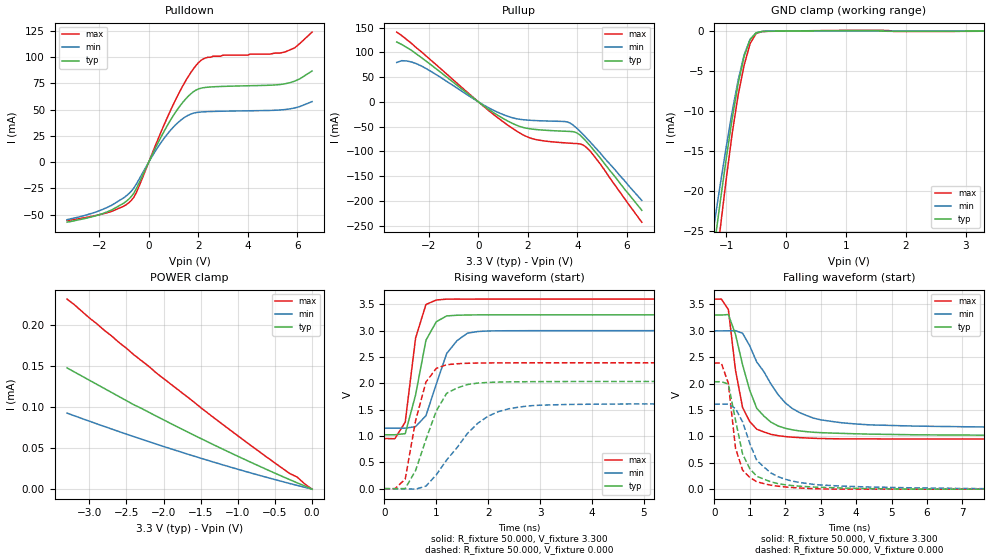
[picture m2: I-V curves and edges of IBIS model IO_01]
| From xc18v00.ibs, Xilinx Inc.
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|   Model IO_01
[Model]   IO_01
Model_type   I/O
Polarity   Inverting
Enable   Active-High
Vinl =   0.800V
Vinh =   2.000V
Vmeas =   1.650V
Cref =  50.000pF
Rref =   1.000M
Vref =  0.000V
C_comp   6.700pF   5.700pF   7.600pF
[Temperature Range]   50.000   100.000   0.000
[Voltage Range]   3.300V   3.000V   3.600V
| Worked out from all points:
|   slope of the pulldown table from 0 to 0.495 V, typ, clamps not added: 20.7 ohm
|   slope of the pullup table from 0 to 0.495 V, typ, clamps not added: 27.8 ohm
|   GND clamp passes 1 mA (typ) near -0.59 V on its own axis
|   rising waveform, R_fixture 50.000, V_fixture 3.300: 20-80 % time 297ps typ, 408ps min, 239ps max; typ from 1.02 V to 3.3 V
|   rising waveform, R_fixture 50.000, V_fixture 0.000: 20-80 % time 469ps typ, 827ps min, 316ps max; typ from 0 V to 2.04 V
|   falling waveform, R_fixture 50.000, V_fixture 3.300: 20-80 % time 642ps typ, 1.14ns min, 392ps max; typ from 3.3 V to 1.02 V
|   falling waveform, R_fixture 50.000, V_fixture 0.000: 20-80 % time 482ps typ, 780ps min, 329ps max; typ from 2.04 V to 0 V
[Pulldown]
| voltage   I(typ)   I(min)   I(max)
-3.3V     -57.2mA    -54.8mA    -55.7mA
-1.7V     -47.57mA   -43.39mA   -48.32mA
-700mV    -32.66mA   -27.57mA   -36.39mA
-500mV    -25.26mA   -20.88mA   -29mA
300mV     14.82mA    11.72mA    17.61mA
900mV     40.85mA    30.95mA    50.29mA
1.6V      62.9mA     44.78mA    81.73mA
2.1V      70.46mA    47.8mA     96.79mA
3V        72.23mA    48.59mA    102mA
5.5V      74.68mA    50.15mA    105mA
5.9V      77.27mA    51.71mA    109mA
6.6V      86.93mA    57.76mA    124mA
[Pullup]
| voltage   I(typ)   I(min)   I(max)
-3.3V     121mA      79.65mA    141mA
-2.9V     110mA      82.69mA    126mA
-2.3V     89.33mA    72.44mA    101mA
300mV     -11.04mA   -8.824mA   -12.73mA
1.5V      -46.27mA   -33.63mA   -57.51mA
1.9V      -52.76mA   -36.44mA   -68.97mA
2.3V      -55.67mA   -37.72mA   -75.79mA
3.7V      -59.69mA   -42.64mA   -83.42mA
4V        -63.32mA   -54.46mA   -84.35mA
4.2V      -71.44mA   -64.25mA   -86.4mA
4.5V      -87.94mA   -80.06mA   -98.42mA
6.6V      -219mA     -199mA     -243mA
[GND_clamp]
| voltage   I(typ)   I(min)   I(max)
-3.3V     -155mA     -140mA     -172mA
-1.2V     -26.97mA   -24.12mA   -31.21mA
-1.1V     -21.35mA   -19.21mA   -24.73mA
-1V       -15.97mA   -14.5mA    -18.53mA
-900mV    -10.95mA   -10.08mA   -12.81mA
-800mV    -6.54mA    -6.125mA   -7.981mA
-700mV    -3.156mA   -2.96mA    -4.255mA
-600mV    -1.062mA   -1.009mA   -1.564mA
-500mV    -216uA     -233uA     -293uA
-400mV    -48.58uA   -49.49uA   -64.66uA
700mV     37.32uA    20.73uA    65.45uA
3.3V      1.628nA    6.9uA      -17.62uA
[POWER_clamp]
| voltage   I(typ)   I(min)   I(max)
-3.3V     148uA      92.8uA     232uA
-2.4V     103uA      64.12uA    164uA
-1.5V     61.88uA    37.81uA    99.54uA
-500mV    19.51uA    11.69uA    31.91uA
-300mV    11.57uA    6.9uA      19.07uA
-200mV    7.689uA    4.565uA    14.73uA
-100mV    4uA        2.274uA    6.481uA
0V        1.628nA    6.511nA    380pA
[Ramp]
| variable   typ   min   max
dV/dt_r   1.221/0.443n   0.967/0.760n   1.433/0.321n
dV/dt_f   1.366/0.616n   1.101/1.088n   1.589/0.410n
R_load = 50.000
[Rising Waveform]
R_fixture = 50.000
V_fixture = 3.300
V_fixture_min = 3.000
V_fixture_max = 3.600
L_fixture = 0.000H
C_fixture = 0.000F
| time   V(typ)   V(min)   V(max)
0s        1.023V     1.148V     951mV
200ps     1.023V     1.148V     949mV
400ps     1.044V     1.148V     1.262V
600ps     1.779V     1.178V     2.859V
800ps     2.818V     1.386V     3.496V
1ns       3.169V     1.985V     3.581V
1.2ns     3.279V     2.566V     3.598V
1.6ns     3.297V     2.951V     3.598V
1.8ns     3.299V     2.983V     3.599V
10ns      3.299V     3V         3.599V
[Rising Waveform]
R_fixture = 50.000
V_fixture = 0.000
V_fixture_min = 0.000
V_fixture_max = 0.000
L_fixture = 0.000H
C_fixture = 0.000F
| time   V(typ)   V(min)   V(max)
0s        0V         0V         0V
200ps     -298uV     110uV      -3.088mV
400ps     1.188mV    -1.293mV   181mV
600ps     345mV      -9.507mV   1.291V
800ps     933mV      48.75mV    2.024V
1ns       1.477V     263mV      2.284V
1.2ns     1.811V     546mV      2.353V
1.8ns     2.004V     1.242V     2.385V
2.6ns     2.029V     1.549V     2.389V
10ns      2.035V     1.611V     2.389V
[Falling Waveform]
R_fixture = 50.000
V_fixture = 3.300
V_fixture_min = 3.000
V_fixture_max = 3.600
L_fixture = 0.000H
C_fixture = 0.000F
| time   V(typ)   V(min)   V(max)
0s        3.3V       3V         3.6V
200ps     3.299V     2.999V     3.602V
400ps     3.309V     3.001V     3.403V
600ps     2.934V     3.003V     2.257V
800ps     2.357V     2.955V     1.547V
1.2ns     1.532V     2.409V     1.136V
1.6ns     1.27V      1.992V     1.039V
2ns       1.154V     1.638V     997mV
3ns       1.071V     1.314V     960mV
10ns      1.023V     1.165V     951mV
[Falling Waveform]
R_fixture = 50.000
V_fixture = 0.000
V_fixture_min = 0.000
V_fixture_max = 0.000
L_fixture = 0.000H
C_fixture = 0.000F
| time   V(typ)   V(min)   V(max)
0s        2.035V     1.611V     2.389V
200ps     2.036V     1.611V     2.391V
400ps     1.992V     1.61V      2.003V
600ps     1.311V     1.528V     779mV
800ps     669mV      1.276V     362mV
1ns       391mV      871mV      223mV
1.2ns     244mV      546mV      141mV
1.8ns     105mV      236mV      56.13mV
2.8ns     40.08mV    90.65mV    9.067mV
10ns      30.04uV    1.855mV    -12.44uV
